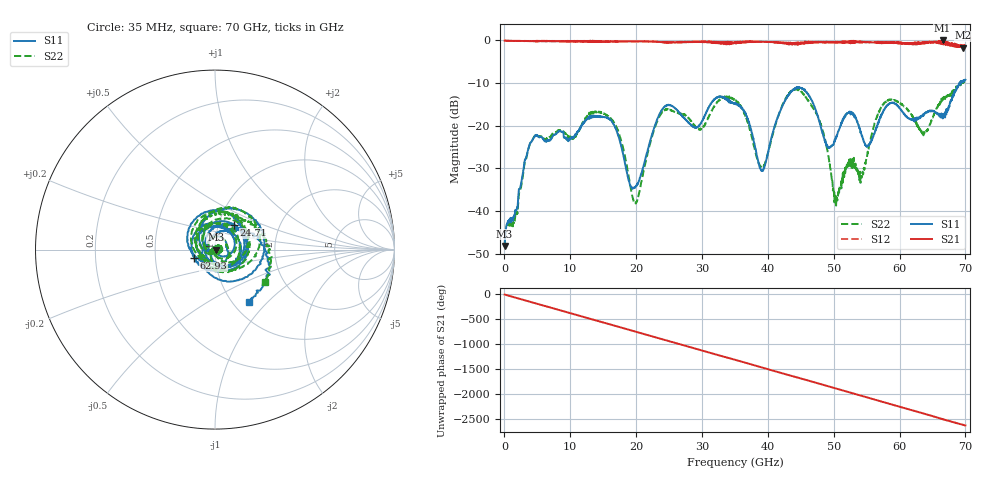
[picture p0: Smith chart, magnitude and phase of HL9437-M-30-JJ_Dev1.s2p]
! 7/27/2020 9:54:21 AM
! H:\PRODUCTION_DATA\TEMP_S2P.S2P
! CHANNEL.1
! TR.MEASUREMENT
! CORRECTED.DATA
# GHZ S RI R 50.0
! FREQ.GHZ  S11RE  S11IM  S21RE  S21IM  S12RE  S12IM  S22RE  S22IM
!; PortSelection: Port_12
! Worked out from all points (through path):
!   2000 points, 35 MHz to 70 GHz, reference 50 ohm
!   highest |S21| = 0.01 dB at 66.53 GHz (marker M1); lowest = -1.7 dB at 69.61 GHz (marker M2)
!   group delay of S21, straight-line fit = 104 ps
!   lowest |S11| = -48.2 dB at 35 MHz (marker M3), VSWR 1.01, Z = 50.4 - j0.118 ohm
!   |S11| at or under -10 dB: start of sweep to 69.12 GHz; 69.17909 GHz to 69.2534 GHz (74.31 MHz wide, 0.107 % of centre)
!   |S22| runs from -48.2 to -9.4 dB; largest |S21 - S12| = 0.083
!   S11 on the Smith chart (normalised r, x): 35 MHz: 1.01, -0.00; 24.71 GHz: 1.18, +0.34; 62.93 GHz: 0.79, -0.08; 70 GHz: 1.18, -0.78
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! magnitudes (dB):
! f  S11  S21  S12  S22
! 35 MHz  -48.2  0.0  0.0  -48.2
! 4.34 GHz  -23.2  -0.1  -0.1  -23.1
! 11.72 GHz  -19.9  -0.2  -0.2  -19.9
! 16.48 GHz  -19.4  -0.3  -0.2  -18.8
! 19.88 GHz  -34.5  -0.2  -0.2  -38.0
! 23.38 GHz  -17.9  -0.3  -0.3  -18.4
! 24.71 GHz  -15.2  -0.5  -0.3  -16.2
! 29.68 GHz  -19.8  -0.3  -0.3  -20.9
! 35.03 GHz  -14.8  -0.5  -0.5  -13.9
! 39.13 GHz  -30.6  -0.3  -0.3  -29.8
! 43.23 GHz  -12.5  -0.6  -0.9  -12.3
! 46.69 GHz  -14.1  -0.5  -0.3  -15.3
! 49.03 GHz  -24.9  -0.4  -0.5  -25.7
! 50.47 GHz  -22.5  -0.5  -0.3  -37.3
! 52.6 GHz  -16.7  -0.5  -0.2  -28.0
! 54.18 GHz  -21.9  -0.3  -0.4  -32.0
! 55.23 GHz  -24.7  -0.4  -0.4  -25.9
! 58.34 GHz  -14.9  -0.6  -0.4  -13.9
! 62.93 GHz  -18.0  -0.6  -0.4  -20.6
! 66.53 GHz  -17.3  0.0  -0.4  -13.4
! 69.61 GHz  -9.5  -1.7  -1.2  -9.9
! 70 GHz  -9.2  -1.3  -1.3  -9.5
